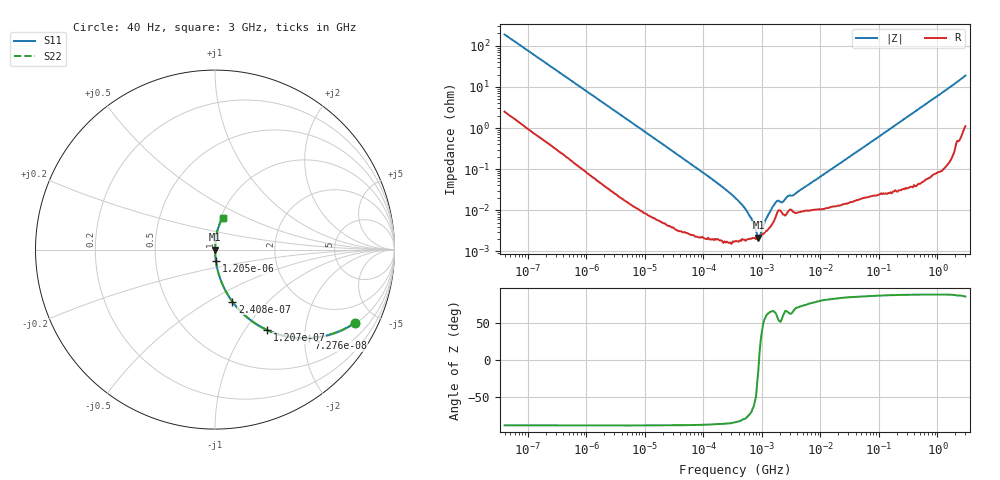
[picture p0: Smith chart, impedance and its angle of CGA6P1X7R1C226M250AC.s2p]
! S-parameter Generated by TDK Corporation
! Copyright(C) 2015 TDK Corporation.
! All Rights Reserved.
! TDK P/N: CGA6P1X7R1C226M250AC (Multilayer Ceramic Chip Capacitors)
! Property: C=22uF
! Size(LxWxT): 3.2x2.5x2.5mm, 0.126x0.098x0.098inches
! Model Type: s2p (Touchstone File Format Version 1.0)
! Frequency: DC=Yes Start=0.00004MHz Stop=3000MHz 396points Log-sweep
! Note: This model was converted from impedance.
! Model Generated on Jun. 23, 2015
! Hash(MD5):
! Port Assignments:
!  1 ---| |--- 2
! Applicable Conditions:
!  Temperature = 25 degC
!  DC Bias Voltage = 0 V
!  Small Signal Operation
! Terms and conditions regarding TDK Simulation Models
! (1)This simulation model is being provided solely for informational purposes. Please refer to the specifications of the products in terms of detailed characteristics of such products.
! (2)In no event shall TDK Corporation of any of its subsidiaries be liable for any loss or damage arising, directly or indirectly,
!  From any information contained in this simulation model, including, but not limited to loss or damages arising from any inaccuracies, omissions or errors in connection with such information.
! (3)Any and all copyrights on this simulation model are owned by TDK Corporation.
!  Duplication or redistribution of this simulation model without prior written permission from TDK Corporation is prohibited.
! (4)This simulation model is subject to any modification or change without any prior notice.
! (5)Neither TDK Corporation nor any of its subsidiaries shall make any warranty, express or implied,
!  Including but not limited to the correctness, implied warranties of merchantability and fitness for a particular purpose with respect to this simulation models.
! (6)The use of this simulation model shall be deemed to have consented to the terms and conditions hereof.
# MHz S MA R 50
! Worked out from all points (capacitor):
!   395 points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, 40 Hz to 3 GHz, reference 50 ohm
!   read as one part in series: C = 21 uF near 41.88 Hz
!   lowest |Z| = 2.16 mohm at 869.6 kHz (marker M1)
!   series resonance near 892.3 kHz, so ESL is about 1.5 nH
!   S11 on the Smith chart (normalised r, x): 40 Hz: 1.05, -3.78; 72.76 Hz: 1.03, -2.10; 120.7 Hz: 1.02, -1.27; 240.8 Hz: 1.01, -0.64; 1.205 kHz: 1.00, -0.13; 3 GHz: 1.02, +0.38
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4e-05  0.8792 -27.7  0.4649 61.5  0.4649 61.5  0.8792 -27.7
7.276073e-05  0.7194 -43.3  0.6856 46.0  0.6856 46.0  0.7194 -43.3
0.0001207144  0.5341 -57.0  0.8389 32.3  0.8389 32.3  0.5341 -57.0
0.0001665986  0.4182 -64.6  0.9033 24.7  0.9033 24.7  0.4182 -64.6
0.0002407527  0.3051 -71.5  0.9486 17.8  0.9486 17.8  0.3051 -71.5
0.0004379335  0.1752 -79.2  0.9825 10.1  0.9825 10.1  0.1752 -79.2
0.000834128  0.09405 -84.0  0.9946 5.4  0.9946 5.4  0.09405 -84.0
0.001205403  0.06563 -85.6  0.9972 3.8  0.9972 3.8  0.06563 -85.6
0.01739424  0.004671 -89.1  0.9999 0.3  0.9999 0.3  0.004671 -89.1
0.1258538  0.0006415 -88.2  1 0.0  1 0.0  0.0006415 -88.2
0.3464102  0.0002037 -85.0  1 0.0  1 0.0  0.0002037 -85.0
0.5488647  9.712e-05 -78.5  1 0.0  1 0.0  9.712e-05 -78.5
0.8696408  2.156e-05 -13.6  1 0.0  1 0.0  2.156e-05 -13.6
1.37789  9.231e-05 65.5  1 -0.0  1 -0.0  9.231e-05 65.5
1.816098  0.0001675 59.2  0.9999 -0.0  0.9999 -0.0  0.0001675 59.2
2.183178  0.0001543 55.6  0.9999 -0.0  0.9999 -0.0  0.0001543 55.6
2.748062  0.0002177 65.7  0.9999 -0.0  0.9999 -0.0  0.0002177 65.7
3.459106  0.0002332 67.3  0.9999 -0.0  0.9999 -0.0  0.0002332 67.3
7.22376  0.000483 78.0  0.9999 -0.0  0.9999 -0.0  0.000483 78.0
150.6385  0.009288 87.9  0.9997 -0.5  0.9997 -0.5  0.009288 87.9
949.3681  0.05726 85.9  0.9976 -3.3  0.9976 -3.3  0.05726 85.9
3000  0.1836 76.1  0.9722 -10.6  0.9722 -10.6  0.1836 76.1
